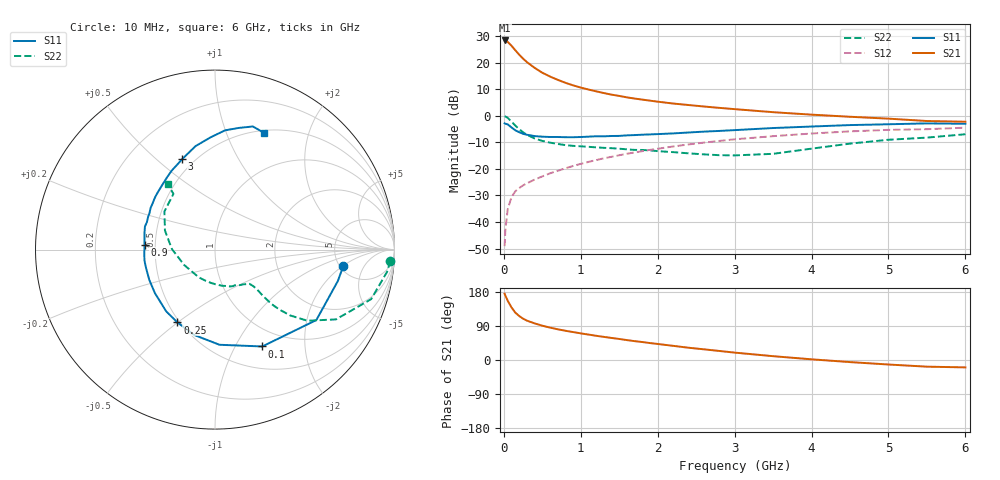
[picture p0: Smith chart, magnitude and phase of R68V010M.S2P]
! SIEMENS Small Signal Semiconductors
! BFR193
! Si NPN RF Bipolar Junction Transistor in SOT23
! VCE = 8 V  IC = 10 mA
! Common Emitter S-Parameters:  May  1996
# GHz  S  MA  R  50
!  f  S11  S21  S12  S22
! GHz  MAG  ANG  MAG  ANG  MAG  ANG  MAG  ANG
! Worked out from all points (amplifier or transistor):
!   36 points, 10 MHz to 6 GHz, reference 50 ohm
!   highest |S21| = 28.3 dB at 10 MHz (marker M1)
!   |S21| within 3 dB of that: start of sweep to 129 MHz
!   unconditionally stable (mu >= 1): 751.9 MHz to 2.056 GHz
!   at 250 MHz: K = 0.63, MSG = 23.9 dB, |S12| = -26.2 dB
!   at 1.4 GHz: K = 1.04, MAG = 10.5 dB, |S12| = -15.5 dB
!   at 6 GHz: K = 0.94, MSG = 1.1 dB, |S12| = -4.5 dB
!   lowest NFmin = 1.30 dB at 450 MHz
!   S11 on the Smith chart (normalised r, x): 10 MHz: 5.33, -2.05; 100 MHz: 0.77, -1.29; 250 MHz: 0.49, -0.50; 900 MHz: 0.44, +0.03; 3 GHz: 0.43, +0.61; 6 GHz: 0.53, +1.37
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0.01  0.7201 -7.4  26.13 175.0  0.0035 85.4  0.9797 -3.7
0.02  0.7066 -14.3  26.09 169.9  0.0071 83.1  0.9664 -7.4
0.05  0.6877 -34.8  24.63 156.5  0.0172 74.4  0.9128 -17.6
0.1  0.6005 -64.0  20.73 138.6  0.0296 64.4  0.7779 -30.0
0.15  0.5308 -87.3  17.04 124.8  0.0378 58.6  0.6495 -37.6
0.2  0.4896 -103.7  14.09 116.0  0.0435 56.5  0.5572 -41.2
0.25  0.4566 -117.3  11.88 109.1  0.0488 55.2  0.4883 -43.0
0.3  0.4386 -128.3  10.23 103.9  0.0534 56.0  0.4383 -43.9
0.4  0.4135 -144.0  7.969 96.6  0.0627 57.6  0.3734 -44.0
0.5  0.4031 -155.3  6.45 90.5  0.072 59.4  0.3355 -43.6
0.6  0.3977 -164.4  5.47 85.5  0.0823 60.7  0.3115 -43.5
0.7  0.3978 -171.4  4.743 81.1  0.0917 61.8  0.2942 -43.7
0.9  0.3935 176.3  3.734 73.7  0.1132 62.6  0.2709 -44.8
1.1  0.4037 166.6  3.113 67.1  0.135 62.6  0.2597 -47.8
1.3  0.4092 158.0  2.672 61.0  0.1579 62.1  0.2485 -51.1
1.6  0.4269 147.3  2.216 52.5  0.1922 60.2  0.2325 -58.6
2.2  0.4644 129.4  1.697 37.4  0.2636 54.6  0.2064 -77.9
3  0.5358 110.0  1.331 19.5  0.3596 44.3  0.1791 -120.2
3.5  0.5865 100.7  1.166 10.1  0.4125 36.9  0.1918 -153.4
4.5  0.6667 85.2  0.956 -5.5  0.5074 22.3  0.2985 159.1
5.5  0.7177 72.9  0.795 -17.6  0.5575 6.9  0.3873 126.7
6  0.7057 67.2  0.771 -19.5  0.5962 2.4  0.4482 125.9
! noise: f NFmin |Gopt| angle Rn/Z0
0.45  1.3  0.22  143  0.11
0.9  1.3  0.34  160  0.11
1.8  2.05  0.54  -153  0.14
